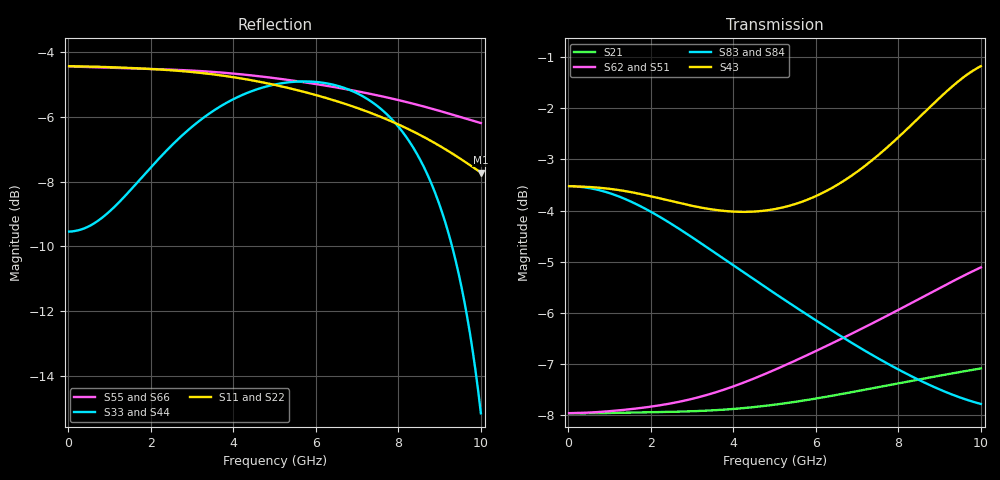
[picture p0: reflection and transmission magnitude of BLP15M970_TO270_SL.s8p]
! Touchstone file from project BLP15M970_TO270
! Exported from HFSS 2017.2.0
! Variables:
!  AirBox_H = 20mm
!  AirBox_L = 30mm
!  AirBox_W = 60mm
!  pcb_h = 502um
# GHZ S MA R 50.000000
! Terminal data exported
! Port[1] = P1_BWT4_9_Rect_T1
! Port[2] = P3_BWT6_9_Rect_T1
! Port[3] = P4_BWT1_Rect_T1
! Port[4] = P6_BWT7_Rect_T1
! Port[5] = P15_BWT10_Rect_T1
! Port[6] = P17_BWT10_Rect_T1
! Port[7] = Box3_T1
! Port[8] = Box2_T1
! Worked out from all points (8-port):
!   450 points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, 22.22 MHz to 10 GHz, reference per port
!   strongest paths, dB at 22.22 MHz, 2.511 GHz, 5.022 GHz, 7.511 GHz, 10 GHz:
!     S43: -3.5, -3.8, -4.0, -2.9, -1.2
!     S83: -3.5, -4.3, -5.6, -6.9, -7.8
!     S84: -3.5, -4.3, -5.6, -6.9, -7.8
!     S62: -8.0, -7.8, -7.1, -6.1, -5.1
!     S51: -8.0, -7.8, -7.1, -6.2, -5.2
!     S21: -8.0, -7.9, -7.8, -7.5, -7.1
!   lowest |S11| = -7.7 dB at 10 GHz (marker M1), VSWR 2.40
!   |S11| at or under -10 dB: nowhere
